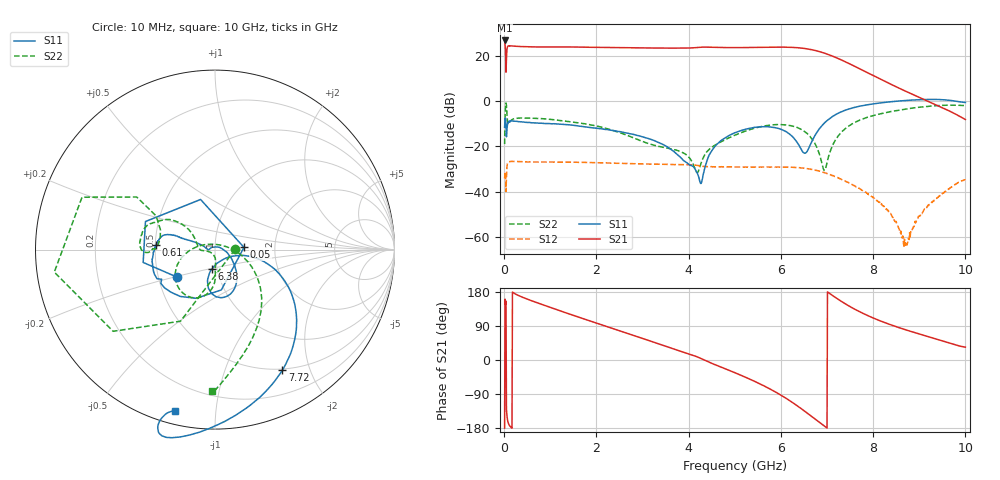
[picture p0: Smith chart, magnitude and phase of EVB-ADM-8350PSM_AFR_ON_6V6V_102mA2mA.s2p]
!Keysight Technologies,N5247B,US58420632,A.15.75.19
!Date: Monday, January 30, 2023 13:29:42
!Correction: S11(C  2-Port  )
!S21(C  2-Port  )
!S12(C  2-Port  )
!S22(C  2-Port  )
!S2P File: Measurements: S11, S21, S12, S22:
# Hz S  dB  R 50
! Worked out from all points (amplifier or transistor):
!   1000 points, 10 MHz to 10 GHz, reference 50 ohm
!   highest |S21| = 26.7 dB at 10 MHz (marker M1)
!   |S21| within 3 dB of that: 69.4 MHz to 1.845 GHz (1.776 GHz wide, 186 % of centre)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
!   unconditionally stable (mu >= 1): start of sweep to 804.8 MHz; 2.291 GHz to 8.566 GHz; 9.857 GHz to end of sweep
!   at 1.67 GHz: K = 0.98, MSG = 25.4 dB, |S12| = -27.1 dB
!   at 5.01 GHz: K = 1.13, MAG = 24.1 dB, |S12| = -29.1 dB
!   at 10 GHz: K = 3.26, MAG = 5.3 dB, |S12| = -34.9 dB
!   S11 on the Smith chart (normalised r, x): 10 MHz: 0.62, -0.20; 50 MHz: 1.38, +0.04; 610 MHz: 0.51, +0.03; 6.38 GHz: 0.94, -0.21; 7.72 GHz: 0.49, -1.60; 10 GHz: 0.06, -0.78
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1e7  -11.61 -144.6  26.66 -179.8  -34.18 75.1  -19.02 0.5
5e7  -15.82 4.4  18.35 -130.8  -33.58 79.5  -1.98 158.5
8e7  -9.76 -126.5  24.10 -162.2  -27.28 39.5  -9.83 160.3
1e8  -9.05 -142.8  24.29 -169.6  -26.85 28.4  -9.93 175.2
1.3e8  -8.84 -153.3  24.26 -175.1  -26.75 19.6  -9.02 -178.8
2.3e8  -8.94 -168.7  24.14 175.2  -26.64 5.4  -7.75 -180.0
6.1e8  -9.68 175.8  23.81 155.7  -26.95 -14.9  -7.63 166.9
1.68e9  -11.24 162.2  23.72 110.4  -27.09 -51.4  -9.88 148.4
2.49e9  -13.48 160.4  23.47 77.6  -27.51 -78.2  -13.88 142.1
3.34e9  -18.22 159.6  23.32 43.0  -27.94 -107.4  -20.00 166.2
4.31e9  -33.09 40.4  23.73 1.5  -28.85 -146.5  -25.32 -87.8
5.01e9  -13.99 -52.2  23.51 -33.9  -29.12 -170.8  -15.04 -90.2
5.44e9  -11.65 -70.6  23.58 -56.9  -29.17 170.2  -11.98 -100.3
5.84e9  -11.64 -88.9  23.71 -81.6  -29.16 150.8  -10.52 -117.0
6.12e9  -13.63 -100.7  23.70 -101.7  -29.16 134.8  -10.59 -132.7
6.38e9  -19.15 -99.1  23.43 -123.0  -29.44 118.0  -11.94 -150.7
6.67e9  -17.90 -15.3  22.58 -149.2  -30.21 97.0  -16.66 -176.7
6.9e9  -10.68 -14.6  21.36 -170.4  -31.39 80.0  -28.48 127.3
7.18e9  -6.11 -30.2  19.24 165.1  -33.40 60.9  -17.31 -9.1
7.72e9  -2.28 -60.8  14.05 126.6  -38.83 31.3  -8.37 -47.0
8.34e9  -0.46 -85.5  7.79 94.7  -48.69 2.9  -4.85 -71.3
1e10  -0.69 -104.0  -8.19 33.9  -34.87 115.8  -2.08 -91.2
